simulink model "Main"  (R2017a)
settings: Solver=VariableStepAuto  StartTime=0.0  StopTime=50  FixedStep=1  RelTol=1e-3
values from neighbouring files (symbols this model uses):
  Hs_swlRange = zeros(states,N)    [run_master.m]
  Hsd_seaRange = zeros(states,N)    [run_master.m]
  Hsd_swlRange = zeros(states,N)    [run_master.m]
  m = 0    [wavespec.m]
  MC_Hs_swl = zeros(states,states,N)    [run_master.m]
  MC_Hsd_sea = zeros(states,states,N)    [run_master.m]
  MC_Hsd_swl = zeros(states,states,N)    [run_master.m]
  MC_Tp_sea = zeros(states,states,N)    [run_master.m]
  MC_Tp_swl = zeros(states,states,N)    [run_master.m]
  MC_u10 = zeros(states,states,N)    [run_master.m]
  MC_u10d = zeros(states,states,N)    [run_master.m]
  n = 0    [wavespec.m]
  Random_Values = generate_random_matrix(seed,SetNumRTs)    [run_master.m]    (also in generate_random_matrix.m = rand(Num_rand,8))
  Tp_seaRange = zeros(states,N)    [run_master.m]
  Tp_swlRange = zeros(states,N)    [run_master.m]
  u10_Range = zeros(states,N)    [run_master.m]
  u10d_Range = zeros(states,N)    [run_master.m]
  v_req_start = 14.5    [run_master.m]
  wpts = [32.8502 121.2880    [run_master.m]
undefined symbols (not defined in the file or in its folder): course_legs, distnm_legs, Hs_seaRange, MC_Hs_sea

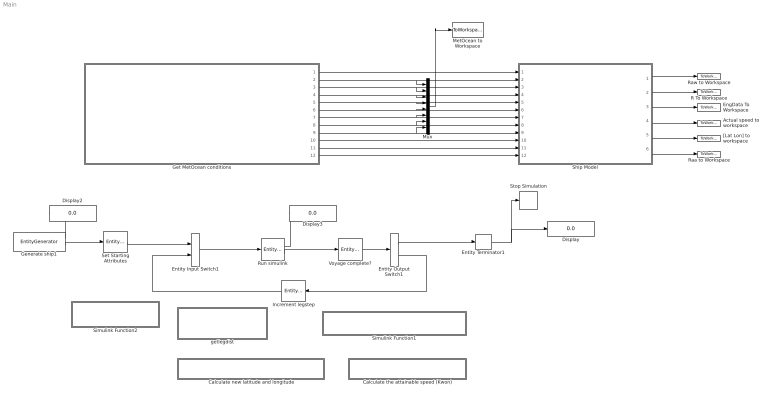
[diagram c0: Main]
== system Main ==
  Actual speed to workspace : ToWorkspace  VariableName=V_act  SaveFormat=Timeseries  SampleTime=-1
  Calculate new latitude and longitude : Subsystem  TreatAsAtomicUnit=on
  Calculate the attainable speed (Kwon) : Subsystem  TreatAsAtomicUnit=on
  Display : Display
  Display2 : Display
  Display3 : Display
  EngData To Workspace : ToWorkspace  VariableName=engroom  SaveFormat=Timeseries  SampleTime=-1
  Entity Input Switch1 : EntityInputSwitch  InputPortMessageModes=m,m  OutputPortMessageModes=m
  Entity Output Switch1 : EntityOutputSwitch  InputPortMessageModes=m  OutputPortMessageModes=m,m  SwitchingCriterion=From attribute  SwitchAttributeName=outputport
  Entity Terminator1 : EntityTerminator  InputPortMessageModes=m  NumberEntitiesArrived=on
  Generate ship1 : EntityGenerator  OutputPortMessageModes=n,m  TimeSource=MATLAB action  IntergenerationTimeAction=|  GenerateEntityAtSimulationStart=off  AttributeName=HsSea_S|HsdSea_S|TpSea_S|HsSwl_S|HsdSwl_S|TpSwl_S|u10_S|u10d_S|speed|outputport|legstep|legdist|leg|course|lat|lon|Hs4k|Hsd4k|Att_speed|Dist_sailed_tot|Dist_sailed_leg|numRTs|Voyage_step  AttributeInitialValue=0|0|0|0|0|0|0|0|15|1|2|1|1|1|1|1|1|1|1|0|0|1|1  NumberEntitiesDeparted=on  EntityType=Structured  EntityTypeName=ship
      | persistent count igt;
      | if isempty(count)
      |     igt=[0 inf];
      |     count=1;
      | end
      | dt=igt(count);
      | count=count+1;
  Get MetOcean conditions : Subsystem  TreatAsAtomicUnit=on
  Increment legstep : EntityServer  InputPortMessageModes=m  OutputPortMessageModes=m  Capacity=1  ServiceTimeValue=0  EntryAction=|
      | %increment the total progress
      | entity.legstep=entity.legstep+1;
  MetOcean to Workspace : ToWorkspace  VariableName=MetOcean  SaveFormat=Timeseries  SampleTime=-1
  Mux : Mux  Inputs=8
  R To Workspace : ToWorkspace  VariableName=R  SaveFormat=Timeseries  SampleTime=-1
  Raa to Workspace : ToWorkspace  VariableName=Raa  SaveFormat=Timeseries  SampleTime=-1
  Raw to Workspace : ToWorkspace  VariableName=Raw  SaveFormat=Timeseries  SampleTime=-1
  Run simulink : EntityServer  InputPortMessageModes=m  OutputPortMessageModes=n,m  Capacity=1  ServiceTimeValue=1  EntryAction=|  NumberEntitiesDeparted=on
      | %take the current leg, and give the vessel its course and the distance of the leg
      | [entity.course,entity.legdist]=readLeg(entity.leg);
      | 
      | %run the ship model, and output the weather states (Markov Chain)
      | [HsSea_S,HsdSea_S,TpSea_S,HsSwl_S,HsdSwl_S,TpSwl_S,hsd4k,hs4k,u10_S,u10d_S] = runSim(entity.legstep,entity.course,entity.speed,entity.leg,...
      |                                                    entity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
  Set Starting Attributes : EntityServer  InputPortMessageModes=m  OutputPortMessageModes=m  Capacity=1  ServiceTimeValue=0  EntryAction=|
      | %Read origin coordinates from waypoints
      | [lat1,lon1,v_req]=SetStart();
      | 
      | %Assign starting coordinates to entity
      | entity.lat=lat1;
      | entity.lon=lon1;
      | 
      | %Assign the intended speed
      | entity.speed=v_req;
  Ship Model : ModelReference  ModelNameDialog=Ship_Model  SimulationMode=Normal  ModelReferenceVersion=1.120
  Simulink Function1 : Subsystem  TreatAsAtomicUnit=on
  Simulink Function2 : Subsystem  TreatAsAtomicUnit=on
  Stop Simulation : Stop
  Voyage complete? : EntityServer  InputPortMessageModes=m  OutputPortMessageModes=m  Capacity=1  ServiceTimeValue=0  EntryAction=|
      | %Check if the entire voyage is complete
      | entity.outputport=checkComplete(entity.leg,entity.legdist,entity.Dist_sailed_leg);
      | 
      | %Check if the current Leg is complete
      | %if entity.Dist_sailed_leg>=entity.legdist
      |  %   entity.leg=entity.leg+1;%start new leg
      |  %   entity.legstep=1; %reset the counter to the new leg
      |   %  entity.Dist_sailed_leg=0; %reset the counter for distance sailed on current leg%
      | %end
  "[Lat Lon] to workspace" : ToWorkspace  VariableName=LatLon  SaveFormat=Timeseries  SampleTime=-1
  getlegdist : Subsystem  TreatAsAtomicUnit=on
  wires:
  Run simulink/1 -> Display3/1
  Generate ship1/2 -> Set Starting Attributes/1
  Entity Input Switch1/1 -> Run simulink/1
  Entity Output Switch1/1 -> Entity Terminator1/1
  Generate ship1/1 -> Display2/1
  Run simulink/2 -> Voyage complete?/1
  Voyage complete?/1 -> Entity Output Switch1/1
  Increment legstep/1 -> Entity Input Switch1/2
  Entity Output Switch1/2 -> Increment legstep/1
  Entity Terminator1/1 -> Stop Simulation/1, Display/1
  Set Starting Attributes/1 -> Entity Input Switch1/1
  Get MetOcean conditions/2(Hs_sea) -> Mux/1, Ship Model/2
  Get MetOcean conditions/10(Course) -> Ship Model/10
  Get MetOcean conditions/7(Tp_swl) -> Mux/6, Ship Model/7
  Ship Model/4 -> Actual speed to workspace/1
  Get MetOcean conditions/3(relD_sea) -> Ship Model/3, Mux/2
  Get MetOcean conditions/4(Tp_sea) -> Mux/3, Ship Model/4
  Ship Model/3 -> EngData To Workspace/1
  Get MetOcean conditions/6(relD_swl) -> Mux/5, Ship Model/6
  Get MetOcean conditions/11(lat) -> Ship Model/11
  Ship Model/2 -> R To Workspace/1
  Get MetOcean conditions/12(lon) -> Ship Model/12
  Mux/1 -> MetOcean to Workspace/1
  Ship Model/1 -> Raw to Workspace/1
  Ship Model/6 -> Raa to Workspace/1
  Get MetOcean conditions/8(u10) -> Ship Model/8, Mux/7
  Get MetOcean conditions/9(relD_u10) -> Ship Model/9, Mux/8
  Get MetOcean conditions/1(vreq) -> Ship Model/1
  Get MetOcean conditions/5(Hs_swl) -> Mux/4, Ship Model/5
  Ship Model/5 -> "[Lat Lon] to workspace"/1

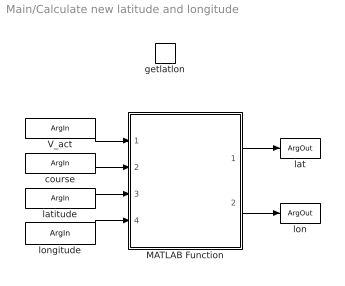
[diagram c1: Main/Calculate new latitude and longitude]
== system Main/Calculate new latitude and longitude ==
  getlatlon : TriggerPort  TriggerType=function-call  IsSimulinkFunction=on  FunctionName=getlatlon  VariantControl=Variant
  MATLAB Function : MATLAB Function  TreatAsAtomicUnit=on
  V_act : ArgIn  DisableCoverage=on  ArgumentName=V_act
  latitude : ArgIn  Port=2  ArgumentName=latitude
  longitude : ArgIn  Port=3  ArgumentName=longitude
  course : ArgIn  Port=4  ArgumentName=course
  lat : ArgOut  DisableCoverage=on  ArgumentName=lat
  lon : ArgOut  Port=2  ArgumentName=lon
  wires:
  V_act/1 -> MATLAB Function/1(V_act)
  MATLAB Function/1(lat_new) -> lat/1
  course/1 -> MATLAB Function/2(Course)
  latitude/1 -> MATLAB Function/3(Lat)
  longitude/1 -> MATLAB Function/4(Lon)
  MATLAB Function/2(lon_new) -> lon/1

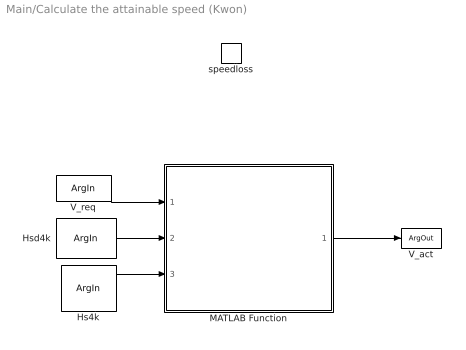
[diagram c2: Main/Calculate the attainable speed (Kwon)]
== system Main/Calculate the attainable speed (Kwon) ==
  speedloss : TriggerPort  TriggerType=function-call  IsSimulinkFunction=on  FunctionName=speedloss  VariantControl=Variant
  MATLAB Function : MATLAB Function  TreatAsAtomicUnit=on
  V_req : ArgIn  DisableCoverage=on  ArgumentName=V_req
  Hsd4k : ArgIn  Port=2  ArgumentName=Hsd4k
  Hs4k : ArgIn  Port=3  ArgumentName=Hs4k
  V_act : ArgOut  DisableCoverage=on  ArgumentName=V_act
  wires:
  MATLAB Function/1(V_act) -> V_act/1
  Hs4k/1 -> MATLAB Function/3(Hs)
  Hsd4k/1 -> MATLAB Function/2(rel_heading)
  V_req/1 -> MATLAB Function/1(V_req)

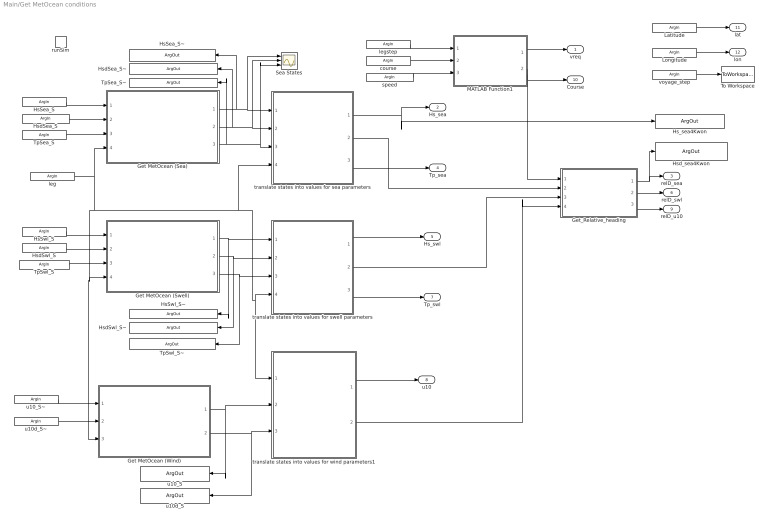
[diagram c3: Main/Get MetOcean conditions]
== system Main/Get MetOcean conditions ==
  runSim : TriggerPort  TriggerType=function-call  IsSimulinkFunction=on  FunctionName=runSim  VariantControl=Variant
  Get MetOcean (Sea) : MATLAB Function  TreatAsAtomicUnit=on
  Get MetOcean (Swell) : MATLAB Function  TreatAsAtomicUnit=on
  Get MetOcean (Wind) : MATLAB Function  TreatAsAtomicUnit=on
  Get_Relative_heading : MATLAB Function  TreatAsAtomicUnit=on
  MATLAB Function1 : MATLAB Function  TreatAsAtomicUnit=on
  Sea States : Scope  NumInputPorts=3
  To Workspace : ToWorkspace  VariableName=voyage_step  SaveFormat=Timeseries  SampleTime=-1
  translate states into values for swell parameters : MATLAB Function  TreatAsAtomicUnit=on
  translate states into values for wind parameters1 : MATLAB Function  TreatAsAtomicUnit=on
  translate states into values for sea parameters : MATLAB Function  TreatAsAtomicUnit=on
  legstep : ArgIn  ArgumentName=legstep
  course : ArgIn  Port=2  ArgumentName=course
  speed : ArgIn  Port=3  ArgumentName=speed
  leg : ArgIn  Port=4  ArgumentName=leg
  HsSwl_S : ArgIn  Port=5  ArgumentName=HsSwl_S
  HsdSwl_S : ArgIn  Port=6  ArgumentName=HsdSwl_S
  TpSwl_S : ArgIn  Port=7  ArgumentName=TpSwl_S
  HsSea_S : ArgIn  Port=8  ArgumentName=HsSea_S
  HsdSea_S : ArgIn  Port=9  ArgumentName=HsdSea_S
  TpSea_S : ArgIn  Port=10  ArgumentName=TpSea_S
  Latitude : ArgIn  Port=11  ArgumentName=Latitude
  Longitude : ArgIn  Port=12  ArgumentName=Longitude
  u10_S~ : ArgIn  Port=13  ArgumentName=u10_S
  u10d_S~ : ArgIn  Port=14  ArgumentName=u10d_S
  voyage_step : ArgIn  Port=15  ArgumentName=voyage_step
  HsSea_S~ : ArgOut  ArgumentName=HsSea_S
  HsdSea_S~ : ArgOut  Port=2  ArgumentName=HsdSea_S
  TpSea_S~ : ArgOut  Port=3  ArgumentName=TpSea_S
  HsSwl_S~ : ArgOut  Port=4  ArgumentName=HsSwl_S
  HsdSwl_S~ : ArgOut  Port=5  ArgumentName=HsdSwl_S
  TpSwl_S~ : ArgOut  Port=6  ArgumentName=TpSwl_S
  Hsd_sea4Kwon : ArgOut  Port=7  ArgumentName=Hsd_sea4Kwon
  Hs_sea4Kwon : ArgOut  Port=8  ArgumentName=Hs_sea4Kwon
  u10_S : ArgOut  Port=9  ArgumentName=u10_S
  u10d_S : ArgOut  Port=10  ArgumentName=u10d_S
  vreq : Outport
  Hs_sea : Outport  Port=2
  relD_sea : Outport  Port=3
  Tp_sea : Outport  Port=4
  Hs_swl : Outport  Port=5
  relD_swl : Outport  Port=6
  Tp_swl : Outport  Port=7
  u10 : Outport  Port=8
  relD_u10 : Outport  Port=9
  Course : Outport  Port=10
  lat : Outport  Port=11
  lon : Outport  Port=12
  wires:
  leg/1 -> Get MetOcean (Sea)/4(leg), Get MetOcean (Wind)/3(leg), Get MetOcean (Swell)/4(leg), translate states into values for wind parameters1/1(leg), translate states into values for swell parameters/4(leg), translate states into values for sea parameters/4(leg)
  Get MetOcean (Sea)/1(Sea_HSS) -> HsSea_S~/1, Sea States/1, translate states into values for sea parameters/1(HsSea_S)
  Get MetOcean (Sea)/2(Sea_HSDS) -> HsdSea_S~/1, Sea States/2, translate states into values for sea parameters/2(HsdSea_S)
  Get MetOcean (Sea)/3(Sea_TPS) -> TpSea_S~/1, Sea States/3, translate states into values for sea parameters/3(TpSea_S)
  translate states into values for sea parameters/1(Hs_sea) -> Hs_sea4Kwon/1, Hs_sea/1
  translate states into values for sea parameters/3(Tp_sea) -> Tp_sea/1
  Get MetOcean (Swell)/2(HSD_S) -> HsdSwl_S~/1, translate states into values for swell parameters/2(HsdSwl_S)
  Get MetOcean (Swell)/3(TM_S) -> TpSwl_S~/1, translate states into values for swell parameters/3(TpSwl_S)
  translate states into values for swell parameters/2(Hsd_swl) -> Get_Relative_heading/3(Hsd_swl)
  Get MetOcean (Swell)/1(HS_S) -> HsSwl_S~/1, translate states into values for swell parameters/1(HsSwl_S)
  translate states into values for swell parameters/1(Hs_swl) -> Hs_swl/1
  translate states into values for swell parameters/3(Tp_swl) -> Tp_swl/1
  MATLAB Function1/1(Vreq) -> vreq/1
  MATLAB Function1/2(Course) -> Get_Relative_heading/1(course), Course/1
  HsSea_S/1 -> Get MetOcean (Sea)/1(Hs_SeS)
  HsdSea_S/1 -> Get MetOcean (Sea)/2(Hsd_SeS)
  TpSea_S/1 -> Get MetOcean (Sea)/3(Tp_SeS)
  TpSwl_S/1 -> Get MetOcean (Swell)/3(Per_S)
  HsdSwl_S/1 -> Get MetOcean (Swell)/2(Head_S)
  HsSwl_S/1 -> Get MetOcean (Swell)/1(Wave_S)
  speed/1 -> MATLAB Function1/3(speed)
  course/1 -> MATLAB Function1/2(course)
  legstep/1 -> MATLAB Function1/1(legstep)
  Latitude/1 -> lat/1
  Longitude/1 -> lon/1
  u10_S~/1 -> Get MetOcean (Wind)/1(windVel_S)
  translate states into values for wind parameters1/1(u10) -> u10/1
  translate states into values for sea parameters/2(Hsd_sea) -> Get_Relative_heading/2(Hsd_sea)
  translate states into values for wind parameters1/2(u10d) -> Get_Relative_heading/4(u10d)
  Get_Relative_heading/3(relD_u10) -> relD_u10/1
  Get_Relative_heading/2(relD_swl) -> relD_swl/1
  Get_Relative_heading/1(relD_sea) -> Hsd_sea4Kwon/1, relD_sea/1
  Get MetOcean (Wind)/1(u10_S) -> u10_S/1, translate states into values for wind parameters1/2(u10_S)
  Get MetOcean (Wind)/2(u10d_S) -> u10d_S/1, translate states into values for wind parameters1/3(u10d_S)
  u10d_S~/1 -> Get MetOcean (Wind)/2(windDir_S)
  voyage_step/1 -> To Workspace/1

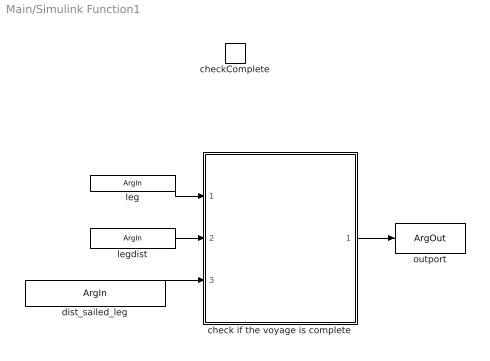
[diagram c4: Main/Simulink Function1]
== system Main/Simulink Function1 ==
  checkComplete : TriggerPort  TriggerType=function-call  IsSimulinkFunction=on  FunctionName=checkComplete  VariantControl=Variant
  check if the voyage is complete : MATLAB Function  TreatAsAtomicUnit=on
  leg : ArgIn  DisableCoverage=on  ArgumentName=leg
  legdist : ArgIn  Port=2  ArgumentName=legdist
  dist_sailed_leg : ArgIn  Port=3  ArgumentName=dist_sailed_leg
  outport : ArgOut  DisableCoverage=on  ArgumentName=outport
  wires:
  leg/1 -> check if the voyage is complete/1(leg)
  check if the voyage is complete/1(outport) -> outport/1
  dist_sailed_leg/1 -> check if the voyage is complete/3(dist_sailed_leg)
  legdist/1 -> check if the voyage is complete/2(legdist)

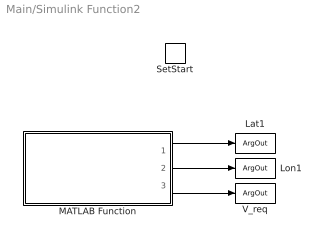
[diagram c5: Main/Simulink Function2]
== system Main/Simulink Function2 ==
  SetStart : TriggerPort  TriggerType=function-call  IsSimulinkFunction=on  FunctionName=SetStart  VariantControl=Variant
  MATLAB Function : MATLAB Function  TreatAsAtomicUnit=on
  Lat1 : ArgOut  DisableCoverage=on  ArgumentName=Lat1
  Lon1 : ArgOut  Port=2  ArgumentName=Lon1
  V_req : ArgOut  Port=3  ArgumentName=V_req
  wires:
  MATLAB Function/2(Lon1) -> Lon1/1
  MATLAB Function/1(Lat1) -> Lat1/1
  MATLAB Function/3(v_req) -> V_req/1

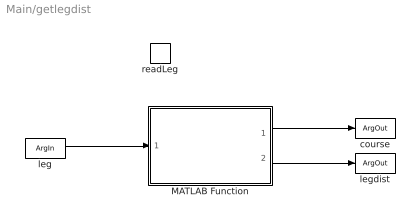
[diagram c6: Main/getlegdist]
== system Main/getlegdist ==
  readLeg : TriggerPort  TriggerType=function-call  IsSimulinkFunction=on  FunctionName=readLeg  VariantControl=Variant
  MATLAB Function : MATLAB Function  TreatAsAtomicUnit=on
  leg : ArgIn  DisableCoverage=on  ArgumentName=leg
  course : ArgOut  DisableCoverage=on  ArgumentName=course
  legdist : ArgOut  DisableCoverage=on  Port=2  ArgumentName=legdist
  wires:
  leg/1 -> MATLAB Function/1(leg)
  MATLAB Function/1(course) -> course/1
  MATLAB Function/2(legdist) -> legdist/1

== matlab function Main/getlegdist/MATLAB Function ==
function [course,legdist] = fcn(leg,distnm_legs,course_legs)
%take in the current leg that the vessel is on, and give the distance for
%that leg, and the course
course=course_legs(leg);
legdist=distnm_legs(leg);
    
end

== matlab function Main/Get MetOcean conditions/translate states into values 
for sea parameters ==
function [Hs_sea, Hsd_sea, Tp_sea] = weatherValues(HsSea_S, HsdSea_S, TpSea_S, leg, Hs_seaRange, Hsd_seaRange, Tp_seaRange)



Hs_sea = Hs_seaRange(HsSea_S, leg);
Hsd_sea = Hsd_seaRange(HsdSea_S, leg);
Tp_sea = Tp_seaRange(TpSea_S, leg);

end

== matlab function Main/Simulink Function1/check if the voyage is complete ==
function outport = fcn(leg,legdist,dist_sailed_leg,distnm_legs)

dist=dist_sailed_leg; %the distance sailed on current leg

if leg == length(distnm_legs) && dist>=(legdist-20) %subtract to avoid errors
    outport=1; %Journey complete
else
    outport=2; %Journey not complete
end

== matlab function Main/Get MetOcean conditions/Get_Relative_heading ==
function [relD_sea, relD_swl, relD_u10] = fcn(course, Hsd_sea, Hsd_swl, u10d)

relD_sea = (Hsd_sea-course);
relD_swl = (Hsd_swl-course);
relD_u10 = (u10d-course);

end

== matlab function Main/Get MetOcean conditions/translate states into values
for swell parameters ==
function [Hs_swl, Hsd_swl, Tp_swl] = weatherValues(HsSwl_S, HsdSwl_S, TpSwl_S, leg, Hs_swlRange, Hsd_swlRange, Tp_swlRange)

Hs_swl = Hs_swlRange(HsSwl_S, leg);
Hsd_swl = Hsd_swlRange(HsdSwl_S, leg);
Tp_swl = Tp_swlRange(TpSwl_S, leg);

end

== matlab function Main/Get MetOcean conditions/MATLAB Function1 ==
function [Vreq, Course]  = fcn(legstep, course, speed)



%pre-allocating as integers to avoid error message
% heading=0;
% period=0;
% Hs=0;

%declare these functions as extrinsic to be able to use them in simulink
%block
% coder.extrinsic('sprintf');
% coder.extrinsic('xlsread');

%If location has changed, then we can change what spreadsheet we look at,
%but for now we use the same spreadsheet

% filename = 'weatherinput.xlsx';
% xlRange = sprintf('B%d:BB%d',legstep,legstep);
% [numw,~] = xlsread(filename,xlRange);

% Reading MetOcean data directly from parameters
Vreq = speed;

Course=course;
% heading=Wave_Heading(legstep); %numw(4);
% period=Wave_Period(legstep); %numw(6);
% Hs=Wave_HS(legstep); %numw(5);


end

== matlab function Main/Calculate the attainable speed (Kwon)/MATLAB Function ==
function V_act = speedloss_Kwon(V_req,rel_heading,Hs, num)
coder.extrinsic('wrapTo180')
%Use Kwons method to estimate the speed loss due to added resistance

%pre allocate values
V_act=0;
V_2=0; %pre allocate the new speed
Bn=0;
Volume_deplacement=0;
C_u=0;
C_beta=0;
C_form=0;
heading_rel=0;

V_1=V_req*0.5144; %Convert the required speed (set speed) from kts to m/s
heading_rel=abs(wrapTo180(rel_heading)); %convert to 0-180 degrees
Volume_deplacement=num(54); %[m^3]
L=num(3); %Use Lwl
C_B=num(8); %block Coefficient



%calculate the current Froude Number
F_n=V_1/((9.81*L)^0.5);

%Get Beaufort scale number from waveheight
if Hs<0.2
    Bn=1;
elseif Hs>=0.2 && Hs<0.5
    Bn=2;
elseif Hs>=0.5 && Hs<1
    Bn=3;
elseif Hs>=1 && Hs<2
    Bn=4;
elseif Hs>2 && Hs<3
    Bn=5;
elseif Hs>3 && Hs<4
    Bn=6;
elseif Hs>4 %&& Hs<5.5
    Bn=7;
else
    disp('Bn is too high for Kwons method')
end
    

%calculate speed reduction coefficient
if C_B>=0.55 && C_B<0.575
    C_u=1.7-(1.4*F_n)-(7.4*(F_n^2));
elseif C_B>=0.575 && C_B<0.625
    C_u=2.2-(2.5*F_n)-(9.7*(F_n^2));
elseif C_B>=0.625 && C_B<0.675
    C_u=2.6-(3.7*F_n)-(11.6*(F_n^2));
elseif C_B>=0.675 && C_B<0.725
    C_u=3.1-(5.3*F_n)-(12.4*(F_n^2));
elseif C_B>=0.725 && C_B<0.775
    C_u=2.4-(10.6*F_n)-(9.5*(F_n^2));
elseif C_B>=0.775 && C_B<0.825
    C_u=2.6-(13.1*F_n)-(15.1*(F_n^2));
else %C_B>=0.825
    C_u=3.1-(18.7*F_n)+(28*(F_n^2));
end

%calculate direction reduction coefficient
if heading_rel>=0 && heading_rel<30 %head sea
    C_beta=1;
elseif heading_rel>=30 && heading_rel<60 %Bow sea
    C_beta=(1.7-0.03*((Bn-4)^2))/2;
elseif heading_rel>=60 && heading_rel<150 %Beam sea
    C_beta=(0.9-0.06*((Bn-6)^2))/2;
else %heading_rel>=150 && heading_rel<180 %Following sea
    C_beta=(0.4-0.03*((Bn-8)^2))/2;
end

%calculate the ship form coefficient
%valid for all ships, exept container ships, in loaded condition
%C_form=(0.5*Bn)+((Bn^(6.5))/((2.7*(Volume_deplacement^(2/3)))));

%valid for container ships in normal condition
C_form=(0.7*Bn)+((Bn^(6.5))/((22*(Volume_deplacement^(2/3)))));

%percentage loss calculated
%percentage_loss=((V_1-V_2)/V_1)*100;





%calculate deltaV/V1*100%
%Delta_V_overV=C_beta*C_u*C_form;
%coefficient=C_form*C_beta*C_u
%calculate actual ship speed in the selected weather [m/s]
% V_2=V_1-((Delta_V_overV)*(V_1/100))
V_2=V_1-((C_beta*C_u*C_form)*(V_1/100));

%calculate the absolute speed loss [m/s]
%delta_V=V_1-V_2



%if the speed loss found is negative, set the speed to the original speed
% This means that the approximate method did not work in this case
% if V_2>=V_1
%     V_2=V_1; 
%     disp('Approximate method not valid')
%     
% end

V_act=V_2/0.5144; % The actual attainable speed in kts
end


% %function V_act = speedloss_Kwon(V_req,rel_heading,Hs, num)
% %Use Kwons method to estimate the speed loss due to added resistance
% 
% V_1=V_req*0.5144; %Convert the required speed (set speed) from kts to m/s
% heading_rel=rel_heading;
% Volume_deplacement=num(54); %[m^3]
% L=num(3); %Use Lwl
% C_B=num(8); %block Coefficient
% 
% 
% %calculate the current Froude Number
% F_n=V_1/((9.81*L)^0.5);
% 
% %Get Beaufort scale number from waveheight
% if Hs<0.2
%     Bn=1;
% elseif Hs>=0.2 && Hs<0.5
%     Bn=2;
% elseif Hs>=0.5 && Hs<1
%     Bn=3;
% elseif Hs>=1 && Hs<2
%     Bn=4;
% elseif Hs>2 && Hs<3
%     Bn=5;
% elseif Hs>3 && Hs<4
%     Bn=6;
% elseif Hs>4 && Hs<5.5
%     Bn=7;
% else
%     disp('Bn is too high for Kwons method')
% end
%     
% 
% %calculate speed reduction coefficient
% if C_B>=0.55 && C_B<0.575
%     C_u=1.7-(1.4*F_n)-(7.4*(F_n^2));
% elseif C_B>=0.575 && C_B<0.625
%     C_u=2.2-(2.5*F_n)-(9.7*(F_n^2));
% elseif C_B>=0.625 && C_B<0.675
%     C_u=2.6-(3.7*F_n)-(11.6*(F_n^2));
% elseif C_B>=0.675 && C_B<0.725
%     C_u=3.1-(5.3*F_n)-(12.4*(F_n^2));
% elseif C_B>=0.725 && C_B<0.775
%     C_u=2.4-(10.6*F_n)-(9.5*(F_n^2));
% elseif C_B>=0.775 && C_B<0.825
%     C_u=2.6-(13.1*F_n)-(15.1*(F_n^2));
% elseif C_B>=0.825
%     C_u=3.1-(18.7*F_n)+(28*(F_n^2));
% end
% 
% %calculate direction reduction coefficient
% if heading_rel>=0 && heading_rel<30 %head sea
%     C_beta=1;
% elseif heading_rel>=30 && heading_rel<60 %Bow sea
%     C_beta=(1.7-0.03*((Bn-4)^2))/2;
% elseif heading_rel>=60 && heading_rel<150 %Beam sea
%     C_beta=(0.9-0.06*((Bn-6)^2))/2;
% elseif heading_rel>=150 && heading_rel<180 %Following sea
%     C_beta=(0.4-0.03*((Bn-8)^2))/2;
% end
% 
% %calculate the ship form coefficient
% %valid for all ships, exept container ships, in loaded condition
% C_form=(0.5*Bn)+((Bn^(6.5))/((2.7*(Volume_deplacement^(2/3)))));
% 
% %calculate deltaV/V1*100%
% %Delta_V_overV=C_beta*C_u*C_form;
% 
% %calculate actual ship speed in the selected weather [m/s]
% % V_2=V_1-((Delta_V_overV)*(V_1/100))
% V_2=V_1-((C_beta*C_u*C_form)*(V_1/100));
% 
% %calculate the absolute speed loss [m/s]
% %delta_V=V_1-V_2
% 
% %percentage loss calculated
% %percentage_loss=((V_1-V_2)/V_1)*100;
% 
% %if the speed loss found is negative, set the speed to the original speed
% % This means that the approximate method did not work in this case
% if V_2>=V_1
%     V_2=V_1; 
%     disp('Approximate method not valid')
%     
% end
% 
% V_act=V_2/0.5144; % The actual attainable speed in kts
% 
% end

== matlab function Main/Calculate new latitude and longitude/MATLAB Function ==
function [lat_new, lon_new] = New_Lat_Lon(V_act,Course,Lat,Lon)

coder.extrinsic('nm2deg')
coder.extrinsic('reckon')
time=1; % one hour time steps

lat_new=0; %preallocate
lon_new=0; %preallocate


distance=V_act*time; %distance sailed [nm]
arc_length=nm2deg(distance); %distance sailed [deg]

[lat_new, lon_new]=reckon(Lat,Lon,arc_length,Course); %new lat and lon


end

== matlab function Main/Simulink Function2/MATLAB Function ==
function [Lat1, Lon1, v_req]= SetStartAttributes(wpts,v_req_start)

start=zeros(1,2);
v_req=0;

start(1,1)=wpts(1,1); %Starting Latitude
start(1,2)=wpts(1,2); %Starting Longitute

Lat1=start(1,1);
Lon1=start(1,2);

v_req=v_req_start;
end

== matlab function Main/Get MetOcean conditions/translate states into values
for wind parameters1 ==
function [u10, u10d] = weatherValues_wind(leg, u10_S, u10d_S, u10_Range, u10d_Range)
                                           

u10 = u10_Range(u10_S, leg);
u10d = u10d_Range(u10d_S, leg);

end

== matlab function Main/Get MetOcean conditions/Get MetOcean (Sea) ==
function [Sea_HSS, Sea_HSDS, Sea_TPS] = MC_Sea (Hs_SeS, Hsd_SeS, Tp_SeS, MC_Hs_sea, MC_Hsd_sea, MC_Tp_sea,leg,Random_Values)

persistent randnum

if isempty(randnum)
    randnum=1;
end

    
% state=0;
% P=0;
% numStates = 0;
r=0;
Sea_HSS = 0;
Sea_HSDS = 0;
Sea_TPS = 0;

%% Run through for each of the separate Markov Chains
for three_mat=1:3
    if three_mat==1
        P = MC_Hs_sea;
%         numStates = length(MC_Hs_sea(:,:,1));
        state = Hs_SeS;
        col=1;
    elseif three_mat==2
        P = MC_Hsd_sea;
%         numStates = length(MC_Hsd_sea(:,:,1));
        state = Hsd_SeS;
        col=2;
    else %three_mat==3
        P= MC_Tp_sea;
%         numStates = length(MC_Tp_sea(:,:,1));
        state = Tp_SeS;
        col=3;
    end
    
    

%% Find accumulative probability for each state, to be able to determine
%starting state

if state == 0 || state > length(P(:,:,1))
        LongRunP1=P(:,:,leg)^1000;
        PStart = zeros(length(LongRunP1),1);
        PStart (1) = LongRunP1(1,1);
            for i =2:length(LongRunP1)
                PStart (i) = PStart(i-1)+ LongRunP1(i,i);
            end

        %%  Determine starting state
        r=Random_Values(randnum,col);
        randnum=randnum+1;
        count = 1;

        if r >=1
            count = length(P(:,:,1));
        else

            while r > PStart (count)
                count = count + 1;
            end
        end

        state = count;

else
%% Find next state from previous

    cum_dist = cumsum(P(state,:,leg));
    
    iter = 0;
    r=Random_Values(randnum,col);
        randnum=randnum+1;
    temp = find(cum_dist>r);

    while isempty(temp) == 1 && iter < 100
        r=Random_Values(randnum,col);
        randnum=randnum+1;
        temp = find(cum_dist>r);
        iter = iter + 1;
    end

    if isempty(temp) == 1
        temp = state;
    end
state = temp(1);
    

end


    if three_mat==1
            Sea_HSS = state;
    elseif three_mat==2
            Sea_HSDS = state;
    else % three_mat==3
            Sea_TPS = state;
    end

end

end

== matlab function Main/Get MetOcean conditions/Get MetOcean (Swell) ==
function [HS_S, HSD_S, TM_S] = MC_Swell (Wave_S, Head_S, Per_S, MC_Hs_swl, MC_Hsd_swl, MC_Tp_swl,leg,Random_Values)

persistent randnum2

if isempty(randnum2)
    randnum2=1;
end

 
% state=0;
% P=0;
% numStates = 0;
r=0;
HS_S = 0;
HSD_S = 0;
TM_S = 0;

%% Run through for each of the separate Markov Chains
for three_mat=1:3
    if three_mat==1
        P = MC_Hs_swl;
%         numStates = length(MC_Hs_swl(:,:,1));
        state = Wave_S;
        col=4;
    elseif three_mat==2
        P = MC_Hsd_swl;
%         numStates = length(MC_Hsd_swl(:,:,1));
        state = Head_S;
        col=5;
    else 
        P= MC_Tp_swl;
%         numStates = length(MC_Tp_swl(:,:,1));
        state = Per_S;
        col=6;
    end


%% Find accumulative probability for each state, to be able to determine 
%  starting state

if state == 0 || state > length(P(:,:,1))
        LongRunP1=P(:,:,leg)^1000;
        PStart = zeros(length(LongRunP1),1);
        PStart (1) = LongRunP1(1,1);
            for i =2:length(LongRunP1)
                PStart (i) = PStart(i-1)+ LongRunP1(i,i);
            end    

%%  Determine starting state
        r=Random_Values(randnum2,col);
        randnum2=randnum2+1;
        count = 1;

        if r ==1
            count = length(P(:,:,1));
        else

            while r > PStart (count)
                count = count + 1;
            end
        end
state = count;

else
%% Find next state from previous

    cum_dist = cumsum(P(state,:,leg));
    iter = 0;
    r=Random_Values(randnum2,col);
    randnum2=randnum2+1;
    temp = find(cum_dist>r);

    while isempty(temp) == 1 && iter < 100
        r=Random_Values(randnum2,col);
        randnum2=randnum2+1;
        temp = find(cum_dist>r);
        iter = iter + 1;
    end

    if isempty(temp) == 1
        temp = state;
    end

%     count = 1;
%     cum_dist = cumsum(P(state,:,leg));
% 
%     if r>=1
%     count = length(cum_dist);
% 
%     else 
%         while r > cum_dist(count)
%             count = count + 1;
%         end
%     end
% 
% % clear Sum_Check
state = temp(1); % Choose first location greater than r

end
    if three_mat==1
            HS_S = state;
    elseif three_mat==2
            HSD_S = state;
    else 
            TM_S = state;
    end


end

end

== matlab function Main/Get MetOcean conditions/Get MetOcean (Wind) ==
function [u10_S, u10d_S] = MC_Wind (windVel_S, windDir_S, leg,  MC_u10, MC_u10d,Random_Values)

persistent randnum3

if isempty(randnum3)
    randnum3=1;
end
% state=0;
% P=0;
% numStates = 0;
r=0;
u10_S = 0;
u10d_S = 0;

%% Run through for each of the separate Markov Chains
for three_mat=1:2
    if three_mat==1
        P = MC_u10;
        state = windVel_S;
        col=7;
    else
        P = MC_u10d;
        state = windDir_S;
        col=8;
    end
%% Find accumulative probability for each state, to be able to determine 
%  starting state

if state == 0 || state > length(P(:,:,1))
        LongRunP1=P(:,:,leg)^1000;
        PStart = zeros(length(LongRunP1),1);
        PStart (1) = LongRunP1(1,1);
            for i =2:length(LongRunP1)
                PStart (i) = PStart(i-1)+ LongRunP1(i,i);
            end    

%%  Determine starting state
        r=Random_Values(randnum3,col);
        randnum3=randnum3+1;
        count = 1;

        if r ==1
            count = length(P(:,:,1));
        else

            while r > PStart (count)
                count = count + 1;
            end
        end
state = count;

else
%% Find next state from previous

    cum_dist = cumsum(P(state,:,leg));
    iter = 0;
    r=Random_Values(randnum3,col);
    randnum3=randnum3+1;
    temp = find(cum_dist>r);

    while isempty(temp) == 1 && iter < 100
         r=Random_Values(randnum3,col);
        randnum3=randnum3+1;
        temp = find(cum_dist>r);
        iter = iter + 1;
    end

    if isempty(temp) == 1
        temp = state;
    end

state = temp(1); % Choose first location greater than r

end
    if three_mat==1
            u10_S = state;
    else
            u10d_S = state;
    end


end

end
